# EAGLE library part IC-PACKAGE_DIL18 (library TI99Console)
Dual In Line
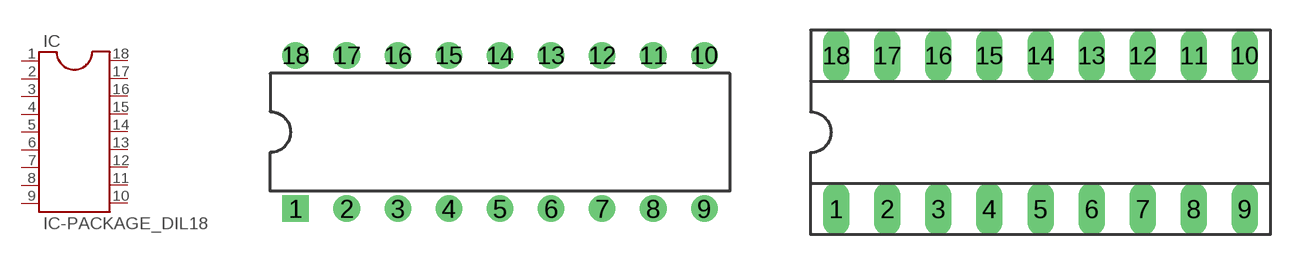
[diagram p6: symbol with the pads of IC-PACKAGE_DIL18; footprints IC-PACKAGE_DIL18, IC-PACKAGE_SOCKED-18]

Designator prefix IC

## IC-PACKAGE_DIL18  [IC-PACKAGE_DIL18]
1  1  pas
2  2  pas
3  3  pas
4  4  pas
5  5  pas
6  6  pas
7  7  pas
8  8  pas
9  9  pas
10  10  pas
11  11  pas
12  12  pas
13  13  pas
14  14  pas
15  15  pas
16  16  pas
17  17  pas
18  18  pas

## IC-PACKAGE_DIL18S  [IC-PACKAGE_SOCKED-18]
Pads as for IC-PACKAGE_DIL18

## Footprint IC-PACKAGE_DIL18 (pad centres in mm)
Dual In Line Package
drill 0.813 square: 1 -10.16,-3.81
drill 0.813: 2 -7.62,-3.81; 3 -5.08,-3.81; 4 -2.54,-3.81; 5 0,-3.81; 6 2.54,-3.81; 7 5.08,-3.81; 8 7.62,-3.81; 9 10.16,-3.81; 10 10.16,3.81; 11 7.62,3.81; 12 5.08,3.81; 13 2.54,3.81; 14 0,3.81; 15 -2.54,3.81; 16 -5.08,3.81; 17 -7.62,3.81; 18 -10.16,3.81

## Footprint IC-PACKAGE_SOCKED-18 (pad centres in mm)
Dual In Line Socked
drill 0.813 long: 1 -10.16,-3.81; 2 -7.62,-3.81; 3 -5.08,-3.81; 4 -2.54,-3.81; 5 0,-3.81; 6 2.54,-3.81; 7 5.08,-3.81; 8 7.62,-3.81; 9 10.16,-3.81; 10 10.16,3.81; 11 7.62,3.81; 12 5.08,3.81; 13 2.54,3.81; 14 0,3.81; 15 -2.54,3.81; 16 -5.08,3.81; 17 -7.62,3.81; 18 -10.16,3.81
